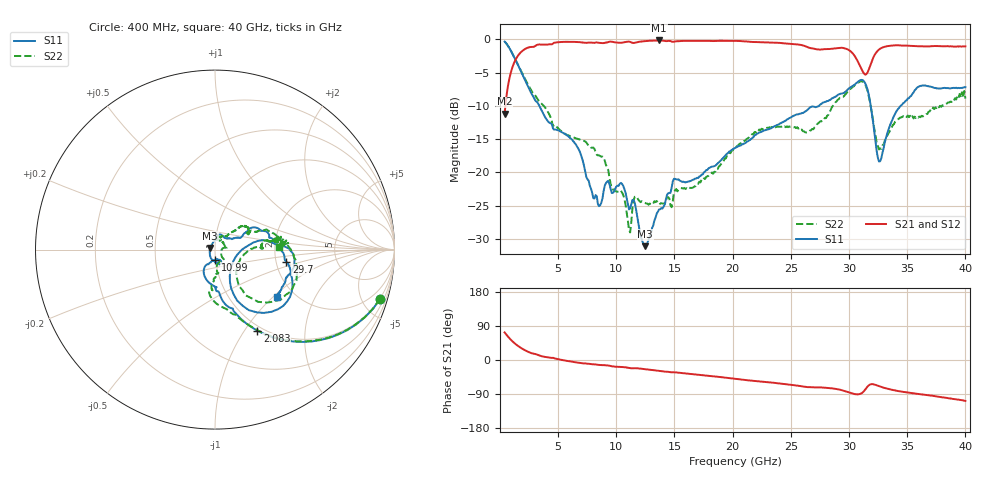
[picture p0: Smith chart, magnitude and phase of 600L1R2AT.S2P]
!  American Technical Ceramics  Date:  10/23/2006
!  One Norden Lane
!  Huntington Station,  NY.  11746-2102
!  Tel:  (631) 622-4700  Fax:  (631) 622-4748
!  Part Number  600L1R2AT Mounting Orientation:  Horizontal
!  Description:  Ultra Low ESR Microwave capacitors
!  Application:  Coupling, Bypass, Tuning, DC Block
!  Filters, Matching
# GHZ S DB R 50
! Freq  |S11|  S11 Ph  |S21|  S21 Ph  |S12|  S12 Ph  |S22|  S22 Ph
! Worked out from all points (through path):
!   401 points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, 400 MHz to 40 GHz, reference 50 ohm
!   highest |S21| = -0.19 dB at 13.67 GHz (marker M1); lowest = -11.2 dB at 400 MHz (marker M2)
!   group delay of S21, straight-line fit = 9 ps
!   lowest |S11| = -31.1 dB at 12.48 GHz (marker M3), VSWR 1.06, Z = 47.4 + j0.881 ohm
!   |S11| at or under -10 dB: 3.384 GHz to 27.42 GHz (24.03 GHz wide, 156 % of centre); 31.86 GHz to 34.44 GHz (2.574 GHz wide, 7.76 % of centre)
!   |S22| runs from -29.0 to -0.4 dB; largest |S21 - S12| = 0.015
!   S11 on the Smith chart (normalised r, x): 400 MHz: 0.94, -6.66; 2.083 GHz: 0.94, -1.15; 10.99 GHz: 1.00, -0.12; 29.7 GHz: 2.28, -0.37; 40 GHz: 1.62, -1.07
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0.4  -0.35 -16.7  -11.17 72.7  -11.13 72.7  -0.36 -16.7
1.093  -2.24 -40.7  -4.11 48.7  -4.07 48.6  -2.23 -40.4
2.083  -5.87 -62.4  -1.55 26.8  -1.51 26.7  -5.72 -61.5
4.261  -12.54 -85.0  -0.76 6.2  -0.73 6.1  -11.37 -94.2
7.033  -17.74 -118.8  -0.48 -8.4  -0.49 -8.7  -15.16 -92.0
8.518  -25.07 -82.3  -0.54 -13.0  -0.56 -13.4  -17.43 -83.0
9.211  -21.37 -69.3  -0.48 -14.2  -0.51 -14.6  -19.22 -83.2
10.993  -24.79 -88.9  -0.37 -20.3  -0.38 -20.4  -27.25 -37.1
11.686  -25.45 -115.5  -0.50 -21.6  -0.51 -21.7  -23.63 5.8
12.478  -31.07 160.6  -0.29 -24.1  -0.30 -24.2  -24.59 19.6
13.666  -25.57 88.6  -0.19 -28.6  -0.21 -28.7  -24.39 45.6
15.052  -20.96 66.6  -0.33 -32.5  -0.36 -32.5  -22.68 73.1
20.2  -16.33 25.1  -0.25 -49.5  -0.28 -49.3  -16.37 43.1
22.675  -13.69 29.4  -0.48 -57.5  -0.50 -57.2  -13.36 37.9
26.833  -10.10 15.3  -1.38 -71.8  -1.39 -71.4  -13.47 27.3
29.704  -7.87 -9.7  -1.41 -82.6  -1.39 -82.3  -8.27 5.4
30.793  -6.35 -26.4  -3.48 -90.5  -3.43 -90.0  -6.51 -14.5
31.486  -7.01 -52.2  -5.25 -74.1  -5.20 -73.5  -7.25 -42.0
32.575  -18.36 -32.7  -1.55 -69.0  -1.50 -68.4  -16.54 -31.0
33.466  -13.19 10.7  -1.00 -77.1  -0.93 -76.6  -13.92 1.2
36.04  -7.07 -5.8  -1.06 -89.9  -0.97 -89.3  -11.61 6.6
40  -7.21 -37.5  -1.08 -107.9  -0.98 -107.3  -8.90 2.0
